(* Logix 5000 AddOnInstructionDefinition export MAG_Yaskawa; software revision 17.00 *)

TYPE Yaskawa_EIP_Servo :   // Yaskawa SigmaLogic Axis Structure v2.4.0
STRUCT
   O : Yaskawa_OUT_to_Servo;
   I : Yaskawa_IN_from_Servo;
   AOI_SB : Yaskawa_AOI_Status_Bits;
END_STRUCT
END_TYPE

TYPE Yaskawa_OUT_to_Servo :   // Structure of data sent out to the Yaskawa SigmaLogic controller v2.4.0
STRUCT
   b00_ServoOn : BOOL;   // Servo On
   b01_Stop : BOOL;   // Stops All Current Motion in Progress
   b02_Home : BOOL;   // Start Homing Process
   b03_MoveStart1 : BOOL;   // Start Current Motion
   b06_SuperImpose : BOOL;
   b07_ServoAlarmReset : BOOL;   // Servo Alarm Reset
   b08_ControllerAlarmReset : BOOL;   // SigmaLogic Alarm Reset
   b09_MoveStart2 : BOOL;   // Start Second Motion (Blended Move)
   b10_MoveAbort : BOOL;   // Abort Current Move
   b11_MovePause : BOOL;   // Pause Current Move
   b12_SeqPause : BOOL;   // Indexing Sequence Pause
   b13_SeqResume : BOOL;   // Indexing Sequence Resume
   b14_SeqCancel : BOOL;   // Indexing Sequence Cancel
   b15_AbsEncoderReset : BOOL;   // Absolute Encoder Reset
   b16_SeqStart : BOOL;   // Start Indexing Sequence
   b17_SeqEditSpeed : BOOL;   // Enter Edit Speed
   b18_SeqEditDistance : BOOL;   // Enter Distance Edit
   b19_PLSEnable : BOOL;   // Enable PLS execution
   b20_PLSActivateOutput1 : BOOL;   // Activate PLS output1 switch logic
   b21_PLSActivateOutput2 : BOOL;   // Activate PLS output2 switch logic
   b22_PLSActivateOutput3 : BOOL;   // Activate PLS output3 switch logic
   b23_PLSActivateOutput4 : BOOL;   // Activate PLS output4 switch logic
   b24_SetClock : BOOL;   // Set the remote controller clock with data provided by the PLC
   RebootController : BOOL;
   UseExternalEncoder : BOOL;   // Use External Encoder when executing MAHSP_Yaskawa
   b32_HeatbeatAnswer : BOOL;   // Heartbeat Answer
   BrakeBypassRequest : BOOL;
   SetFwdTorqueLimit : BOOL;
   SetRevTorqueLimit : BOOL;
   TorqueLimit : DINT;
   TorqueRamp : DINT;
   HomeMethod : INT;
   HomeSpeed : DINT;
   HomeAccDec : DINT;   // Home Move Acceleration/Deceleration Rate
   HomeBackOffDistance : DINT;
   HomeCreepSpeed : DINT;
   HomeCreepDistanceLimit : DINT;
   HomeCreepTimeLimit : DINT;
   HomeOffsetDistance : DINT;
   HomeOffsetSpeed : DINT;
   HomePostion : DINT;
   HomeTorque : DINT;
   HomeInputNo : DINT;
   HomeApproachTimeLimit : DINT;
   HomeApproachDistLimit : DINT;
   HomeDirection : INT;
   HomeSwitchMode : INT;
   MoveType : INT;
   MoveDirection : INT;
   MoveAccel1 : DINT;
   MoveAccel2 : DINT;
   MoveDecel1 : DINT;
   MoveDecel2 : DINT;
   MoveSpeed1 : DINT;
   MoveSpeed2 : DINT;
   MoveDistance1 : DINT;
   MoveDistance2 : DINT;
   MovePosition1 : DINT;
   MovePosition2 : DINT;
   RegistrationDistance : DINT;
   GearNumerator : DINT;
   GearDenominator : DINT;
   SuperImposeDistance : DINT;
   Resolution : INT;
   RegistrationDirection : INT;
   TuningLevel : INT;
   SequenceStep : INT;   // Staring Sequence Step Number
   SequenceEditStep : INT;   // Sequence Step Number to Edit
   FlagCommandBits1 : DINT;   // Flag Commands. 1..64 are General Flags, Bits 0..31 correspond to Flag 1..32
   FlagCommandBits2 : DINT;   // Flag Commands cont. 1..64 are General Flags, Bits 0..31 correspond to Flag 33..64
   DigitalOutCommandBits : DINT;   // Digital Output commands. Bits 0-7 correspond to CN13 Digital Outputs 0-7, used as Flag 73-80. Bits 8-10 correspond to CN1 Digital Outputs 0-2 used as Flag 88-90"
   SequenceEditSpeed : DINT;
   SequenceEditDistance : DINT;
   FeedRateOverride : INT;
   HSI_Enable : BOOL;
   HSI_MoveMode : BOOL;   // 0=Relative; 1=Moves per Cycle
   HSI_CalcMethod : BOOL;   // 0=Accel/Decel; 1=Time
   HSI_MoveDirection : BOOL;   // 0 = Negative; 1 = Positive
   HSI_TriggerFlag : INT;
   HSI_MovingFlag : INT;
   HSI_DwellingFlag : INT;
   HSI_DoneFlag : INT;
   HSI_MoveType : INT;   // 0=Single; 1=Repeat; 2=Repeat "x" times
   HSI_RepeatNumber : INT;
   HSI_Distance : DINT;
   HSI_Speed : DINT;
   HSI_Accel : DINT;
   HSI_MoveTime : DINT;
   HSI_DwellTime : DINT;
   PLS_OutputFlag1 : INT;
   PLS_OutputFlag2 : INT;
   PLS_OutputFlag3 : INT;
   PLS_OutputFlag4 : INT;
   PLS_OnPosition1 : DINT;
   PLS_OffPosition1 : DINT;
   PLS_OnPosition2 : DINT;
   PLS_OffPosition2 : DINT;
   PLS_OnPosition3 : DINT;
   PLS_OffPosition3 : DINT;
   PLS_OnPosition4 : DINT;
   PLS_OffPosition4 : DINT;
   PLS_OnCompensation1 : INT;
   PLS_OffCompensation1 : INT;
   PLS_OnCompensation2 : INT;
   PLS_OffCompensation2 : INT;
   PLS_OnCompensation3 : INT;
   PLS_OffCompensation3 : INT;
   PLS_OnCompensation4 : INT;
   PLS_OffCompensation4 : INT;
   RTC_Year : INT;
   RTC_Month : INT;
   RTC_Day : INT;
   RTC_Hour : INT;
   RTC_Min : INT;
   RTC_Sec : INT;
   StopDecel : DINT;
   AnalogOutput : INT;   // CN13, AO_01 [mV]
END_STRUCT
END_TYPE

TYPE Yaskawa_AOI_Status_Bits :   // Internal bits used to interlock Yaskawa AOI execution. v2.4.0
STRUCT
   MAM : BOOL;   // Move AOI Active
   MAJ : BOOL;   // Jog AOI Active
   MAB : BOOL;   // Blending AOI Active
   MAG : BOOL;   // Gearing AOI Active
   MAHSP : BOOL;   // Home SetPoint AOI Active
   MAH : BOOL;   // Homing AOI Active
   MSQE : BOOL;   // Sequence Edit AOI Active
   MSQR : BOOL;   // Sequence Run AOI Active
   MHSI : BOOL;   // High Speed Index AOI Active
   MSO : BOOL;   // Servo On
   MSF : BOOL;   // Servo Off
   MAFR : BOOL;   // Fault Reset
   MAS : BOOL;   // Servo Abort
   MTRQ : BOOL;   // Torque Mode Active
   MPLS : BOOL;   // PLS Active
   MCLK : BOOL;   // SetClock Active
   MSTL : BOOL;   // Set Torque Limit Active
   AOI_Permissive : BOOL;   // Permissive to Execute an AOI
END_STRUCT
END_TYPE

TYPE Yaskawa_IN_from_Servo :   // Structure of data coming from the Yaskawa SigmaLogic controller. v2.4.0
STRUCT
   AlarmText : STRING;   // ServoPack Alarm Code plus Text Description
   b00_Heartbeat : BOOL;
   b01_Alarm : BOOL;   // ServoPack Alarm
   b02_Warning : BOOL;   // ServoPack Warning
   b03_Ready : BOOL;   // ServoPack Ready
   b04_Enabled : BOOL;   // ServoPack Enabled ("Servo On")
   b05_StopComplete : BOOL;
   b06_HomeComplete : BOOL;
   b07_HomeBusy : BOOL;
   b08_HomeActive : BOOL;
   b09_HomeAborted : BOOL;
   b10_HomeError : BOOL;
   b11_MoveAbsComplete : BOOL;
   b12_MoveAbsBusy : BOOL;
   b13_MoveAbsActive : BOOL;
   b14_MoveAbsAborted : BOOL;
   b15_MoveAbsError : BOOL;
   b16_MoveRelComplete : BOOL;
   b17_MoveRelBusy : BOOL;
   b18_MoveRelActive : BOOL;
   b19_MoveRelAborted : BOOL;
   b20_MoveRelError : BOOL;
   b21_JogAtSpeed : BOOL;
   b22_JogBusy : BOOL;
   b23_JogActive : BOOL;
   b24_JogAborted : BOOL;
   b25_JogError : BOOL;
   b26_GearInSync : BOOL;
   b27_GearBusy : BOOL;
   b28_GearActive : BOOL;
   b29_GearAborted : BOOL;
   b30_GearError : BOOL;
   b32_MoveSuperComplete : BOOL;
   b33_MoveSuperBusy : BOOL;
   b34_MoveSuperActive : BOOL;
   b35_MoveSuperAborted : BOOL;
   b36_MoveSuperError : BOOL;
   b37_PowerCycleRequired : BOOL;
   b38_MoveBlend1Complete : BOOL;
   b39_MoveBlend1Busy : BOOL;
   b40_MoveBlend1Active : BOOL;
   b41_MoveBlend1Abort : BOOL;
   b42_MoveBlend1Error : BOOL;
   b43_MoveBlend2Complete : BOOL;
   b44_MoveBlend2Busy : BOOL;
   b45_MoveBlend2Active : BOOL;
   b46_MoveBlend2Abort : BOOL;
   b47_MoveBlend2Error : BOOL;
   b48_RegComplete : BOOL;
   b49_RegBusy : BOOL;
   b50_RegActive : BOOL;
   b51_RegAborted : BOOL;
   b52_RegError : BOOL;
   b53_ResetAbsEncoderActive : BOOL;
   b54_ResetAbsEncoderBusy : BOOL;
   b55_ResetAbsEncoderDone : BOOL;
   b56_ResetAbsEncoderError : BOOL;
   b57_SeqRunning : BOOL;
   b58_RegSensorNotReached : BOOL;
   b59_SeqEditError : BOOL;
   b60_SeqEditDone : BOOL;
   b61_TorqueAtTorque : BOOL;
   b62_TorqueBusy : BOOL;
   b63_TorqueActive : BOOL;
   b64_TorqueAborted : BOOL;
   b65_TorqueError : BOOL;
   b66_ControllerAlarm : BOOL;
   b67_ApplicationError : BOOL;
   b68_AxisAtStandStill : BOOL;
   b69_TestModeActive : BOOL;
   b70_ServoParamsOK : BOOL;
   b71_SetFwdTorqueLimitDone : BOOL;
   b72_SetRevTorqueLimitDone : BOOL;
   Position : DINT;
   Speed : DINT;
   Torque : DINT;
   HomeErrorID : INT;
   MoveAbsErrorID : INT;
   MoveRelErrorID : INT;
   JogErrorID : INT;
   GearErrorID : INT;
   MoveSuperErrorID : INT;
   ServoAlarmID : INT;
   ServoWarningID : INT;
   ControllerAlarmID : DINT;
   AxisGenAlarmID : DINT;
   MoveBlend1ErrorID : INT;
   MoveBlend2ErrorID : INT;
   ResetAbsEncoderErrorID : INT;
   FunctionBlockErrorID : INT;
   TorqueErrorID : INT;
   RegErrorID : INT;
   SeqCurrentStep : INT;
   FlagStatusBit1 : DINT;   // Flag Status. 1..64 are General Flags, Bits 0..31 correspond to Flag 1..32
   FlagStatusBit2 : DINT;   // Flag Status cont. 1..64 are General Flags, Bits 0..31 correspond to Flag 33..64
   IOStatusBits : DINT;   // Digital IO Status. Bits 0-7, CN13 Inputs 0-7, Used as Flag 65-72. Bits 8-15, CN13 Outputs 0-7, Used as Flag 73-80. Bits 16-22, CN1 Inputs 0-6, Used as Flag 81-87. Bits 23-25, CN1 Outputs 0-4, Used as Flag 88-92.
   HSI_Moving : BOOL;
   HSI_Dwelling : BOOL;
   HSI_Done : BOOL;
   HSI_Busy : BOOL;
   HSI_Error : BOOL;
   HSI_ErrorCode : INT;
   PLS_Running : BOOL;
   PLS_SwitchStatus1 : BOOL;
   PLS_SwitchStatus2 : BOOL;
   PLS_SwitchStatus3 : BOOL;
   PLS_SwitchStatus4 : BOOL;
   PLS_Busy : BOOL;
   PLS_Error : BOOL;
   PLS_ErrorCode : INT;
   SetClock_Done : BOOL;
   SetClock_Busy : BOOL;
   SetClock_Error : BOOL;
   SetClock_ErrorID : INT;
   SoftwareVersion : DINT;
   FirmwareVersion : DINT;
   CommandedPos : DINT;
   CommandedPosNonCyc : DINT;
   CommandedSpeed : DINT;
   Clock_Year : INT;
   Clock_Month : INT;
   Clock_Day : INT;
   Clock_Hour : INT;
   Clock_Minute : INT;
   Clock_Second : INT;
   AnalogInput : REAL;   // CN13, AI_01 [v]
   BrakeBypassActive : BOOL;
   ForwardTorqueLimit : DINT;
   ReverseTorqueLimit : DINT;
END_STRUCT
END_TYPE

ADD_ON_INSTRUCTION MAG_Yaskawa   (* revision 2.4 0, vendor Yaskawa America, Inc., ExecuteEnableInFalse *)
// Motion Axis Gear
// Revision note:
// 2.4.0: No functional change
// 2.3.1: No functional change
// 2.3.0: Fixed bug with exiting MAG properly. Needed to clear MoveType as part of the stopping process not after it was done.
// 2.0.0: Improved output operation and error code reporting. Improved interlocking with embedded code.
// 1.2.0: No functional change.
// Initial Release 9/10/2014
// Help:
// This AOI moves a servo axis in direct proportion to the external encoder at a specified gear ratio. If desired, Superimposed moves may be enabled and executed on top of the gearing motion to adjust the servo position with respect to the external encoder. Acceleration and deceleration is performed at a fixed rate and not over any particular external encoder travel distance. The distance traveled during acceleration will depend on the rate/ratio specified and the current speed of the external encoder. Gear ratio is specified as Slave_Counts/Master_Counts where the values are both DINTs.
VAR_IN_OUT
   Axis : Yaskawa_EIP_Servo; {required}
END_VAR
VAR_INPUT
   Direction : INT; {required}   // 0 = slave axis moves in the same direction as the master axis 1 = slave axis moves in the opposite direction of the master axis. 2 = slave axis reverses from its current or previous direction 3 = slave axis continues in its current or previous direction
   Slave_Counts : DINT; {required}   // Gear Ratio Numerator
   Master_Counts : DINT; {required}   // Gear Ratio Denominator
   Accel_Rate : REAL; {required}   // Acceleration for the Gearing IN [unit/s/s]
   Decel_Rate : REAL; {required}   // Deceleration for the Gearing OUT [unit/s/s]
   SuperUse : INT; {required}   // 0 = Do Not Use Superimpose on Gear 1 = Use SuperImpose on Gear .
   SuperStart : BOOL; {required}   // Signal (pulse) that Starts the SuperImposed Move
   SuperSpeed : REAL; {required}   // Commanded Speed for the SuperImposed Move [unit/s]
   SuperAccel : REAL; {required}   // Acceleration for the SuperImposed Move [unit/s/s]
   SuperDecel : REAL; {required}   // Deceleration for the SuperImposed Move [unit/s/s]
   SuperDistance : REAL; {required}   // Distance (Relative) for the SuperImposed Move [unit/s/s]
END_VAR
VAR_OUTPUT
   EN : BOOL; {visible}   // The AOI is Active
   DN : BOOL; {visible}   // Servo and External Gearing in Sync.
   IP : BOOL; {visible}   // Gearing is In Process
   ER : BOOL; {visible}   // Gearing Motion Error
   SDN : BOOL; {visible}   // SuperImposed Move is Finished
   SIP : BOOL; {visible}   // SuperImposed Move is In Process
   SER : BOOL; {visible}   // SuperImposed Move Error
   FLT_RDY : BOOL; {visible}   // The Servo is Not Ready
   FLT_BSY : BOOL; {visible}   // There is another AOI Active for this Axis
   GearErrorCode : INT; {visible}   // Gearing Error Code
   SuperErrorCode : INT; {visible}   // Move Superimposed Error Code
END_VAR
VAR
   AOI_ON_LOCAL : BOOL;
   db90 : BOOL;   // Shot90
   ScaleFactor : DINT;
   Execute_OS : BOOL;
   Stopping : BOOL;
   Finished : BOOL;   // Function is finished
END_VAR

ROUTINE EnableInFalse   (* ladder *)
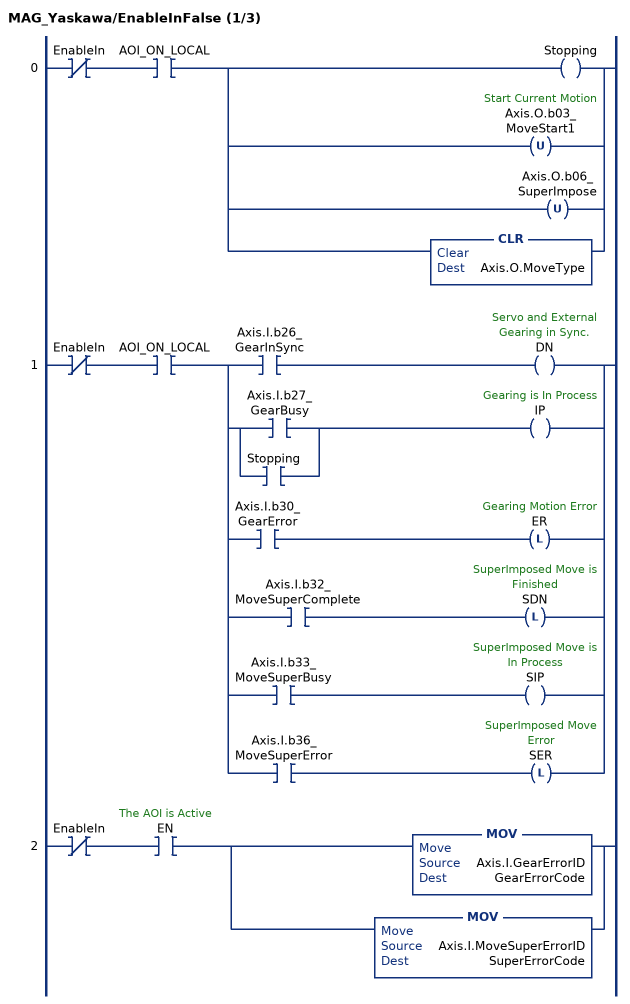
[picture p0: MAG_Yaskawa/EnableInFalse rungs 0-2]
   0: XIO(EnableIn)XIC(AOI_ON_LOCAL)[OTE(Stopping) ,OTU(Axis.O.b03_MoveStart1) ,OTU(Axis.O.b06_SuperImpose) ,CLR(Axis.O.MoveType) ];
   1: XIO(EnableIn)XIC(AOI_ON_LOCAL)[XIC(Axis.I.b26_GearInSync) OTE(DN) ,[XIC(Axis.I.b27_GearBusy) ,XIC(Stopping) ] OTE(IP) ,XIC(Axis.I.b30_GearError) OTL(ER) ,XIC(Axis.I.b32_MoveSuperComplete) OTL(SDN) ,XIC(Axis.I.b33_MoveSuperBusy) OTE(SIP) ,XIC(Axis.I.b36_MoveSuperError) OTL(SER) ];
   2: XIO(EnableIn)XIC(EN)[MOV(Axis.I.GearErrorID,GearErrorCode) ,MOV(Axis.I.MoveSuperErrorID,SuperErrorCode) ];
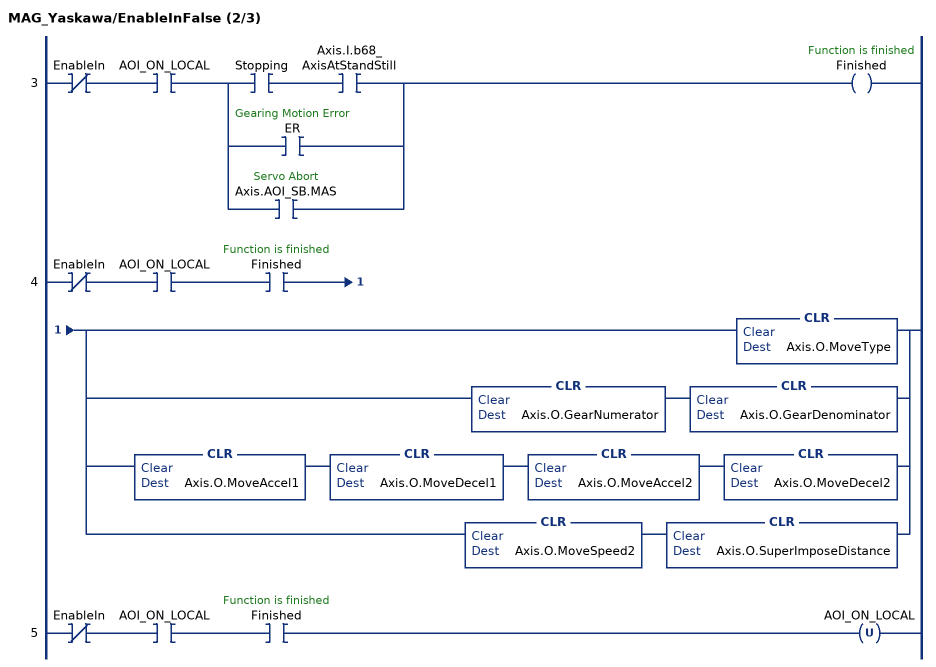
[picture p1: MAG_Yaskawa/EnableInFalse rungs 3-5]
   3: XIO(EnableIn)XIC(AOI_ON_LOCAL)[XIC(Stopping) XIC(Axis.I.b68_AxisAtStandStill) ,XIC(ER) ,XIC(Axis.AOI_SB.MAS) ]OTE(Finished);
   4: XIO(EnableIn)XIC(AOI_ON_LOCAL)XIC(Finished)[CLR(Axis.O.MoveType) ,CLR(Axis.O.GearNumerator) CLR(Axis.O.GearDenominator) ,CLR(Axis.O.MoveAccel1) CLR(Axis.O.MoveDecel1) CLR(Axis.O.MoveAccel2) CLR(Axis.O.MoveDecel2) ,CLR(Axis.O.MoveSpeed2) CLR(Axis.O.SuperImposeDistance) ];
   5: XIO(EnableIn)XIC(AOI_ON_LOCAL)XIC(Finished)OTU(AOI_ON_LOCAL);
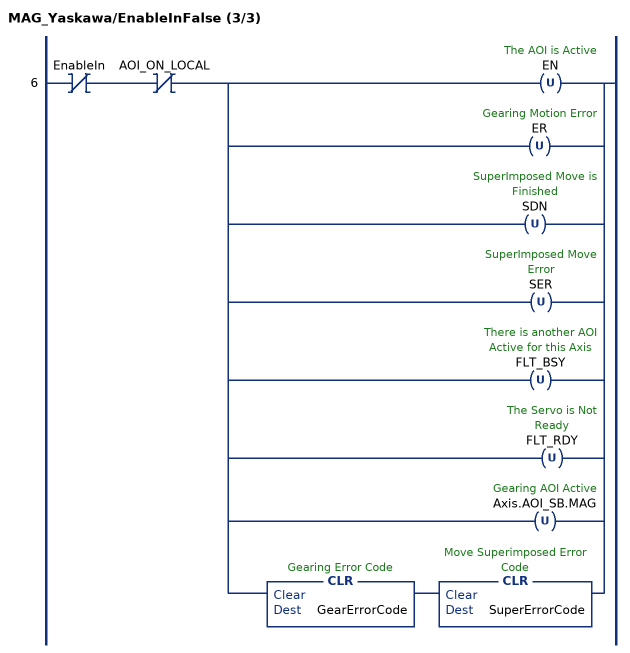
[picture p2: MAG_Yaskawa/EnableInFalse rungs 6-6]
   6: XIO(EnableIn)XIO(AOI_ON_LOCAL)[OTU(EN) ,OTU(ER) ,OTU(SDN) ,OTU(SER) ,OTU(FLT_BSY) ,OTU(FLT_RDY) ,OTU(Axis.AOI_SB.MAG) ,CLR(GearErrorCode) CLR(SuperErrorCode) ];
END_ROUTINE

ROUTINE Logic   (* ladder *)
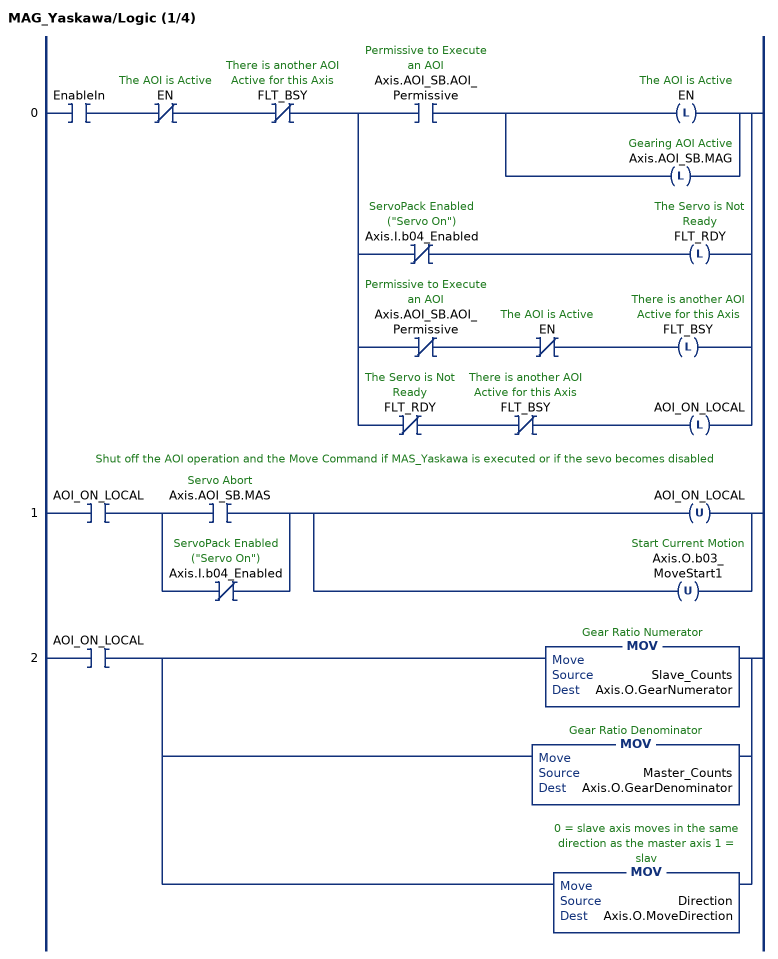
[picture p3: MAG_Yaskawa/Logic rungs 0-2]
   0: XIC(EnableIn)XIO(EN)XIO(FLT_BSY)[XIC(Axis.AOI_SB.AOI_Permissive) [OTL(EN) ,OTL(Axis.AOI_SB.MAG) ] ,XIO(Axis.I.b04_Enabled) OTL(FLT_RDY) ,XIO(Axis.AOI_SB.AOI_Permissive) XIO(EN) OTL(FLT_BSY) ,XIO(FLT_RDY) XIO(FLT_BSY) OTL(AOI_ON_LOCAL) ];
   // Shut off the AOI operation and the Move Command if MAS_Yaskawa is executed or if the sevo becomes disabled
   1: XIC(AOI_ON_LOCAL)[XIC(Axis.AOI_SB.MAS) ,XIO(Axis.I.b04_Enabled) ][OTU(AOI_ON_LOCAL) ,OTU(Axis.O.b03_MoveStart1) ];
   2: XIC(AOI_ON_LOCAL)[MOV(Slave_Counts,Axis.O.GearNumerator) ,MOV(Master_Counts,Axis.O.GearDenominator) ,MOV(Direction,Axis.O.MoveDirection) ];
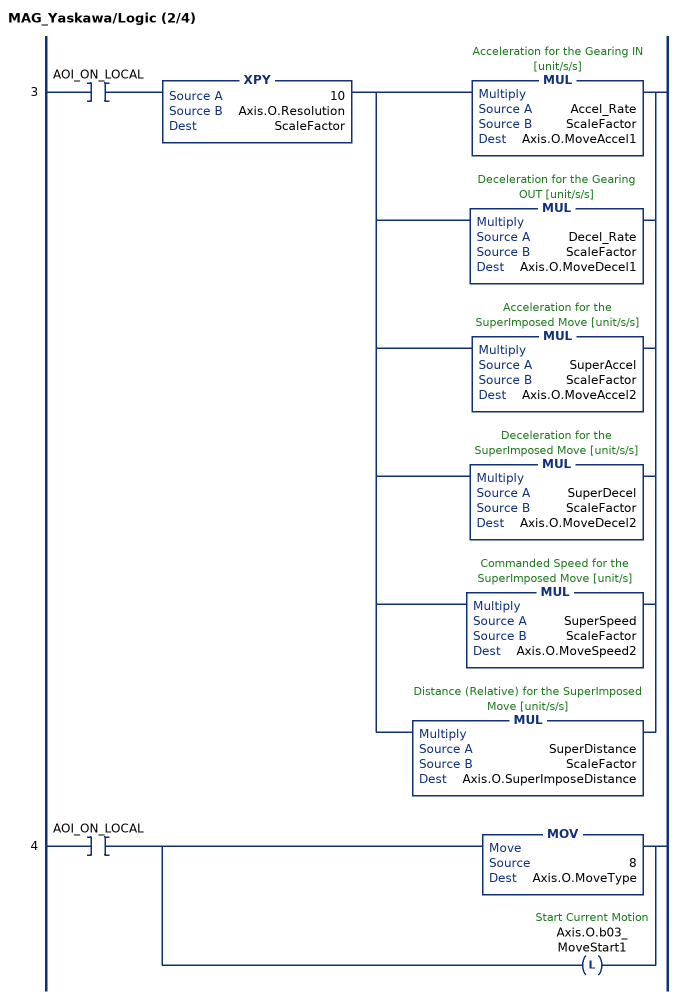
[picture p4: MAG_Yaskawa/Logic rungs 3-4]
   3: XIC(AOI_ON_LOCAL)XPY(10,Axis.O.Resolution,ScaleFactor)[MUL(Accel_Rate,ScaleFactor,Axis.O.MoveAccel1) ,MUL(Decel_Rate,ScaleFactor,Axis.O.MoveDecel1) ,MUL(SuperAccel,ScaleFactor,Axis.O.MoveAccel2) ,MUL(SuperDecel,ScaleFactor,Axis.O.MoveDecel2) ,MUL(SuperSpeed,ScaleFactor,Axis.O.MoveSpeed2) ,MUL(SuperDistance,ScaleFactor,Axis.O.SuperImposeDistance) ];
   4: XIC(AOI_ON_LOCAL)[MOV(8,Axis.O.MoveType) ,OTL(Axis.O.b03_MoveStart1) ];
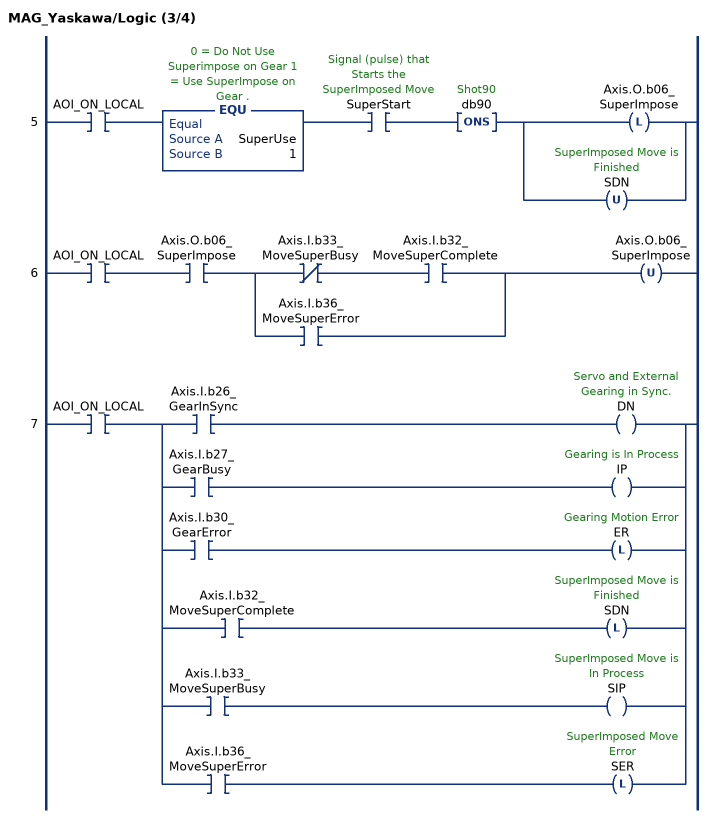
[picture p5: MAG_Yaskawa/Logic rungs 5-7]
   5: XIC(AOI_ON_LOCAL)EQU(SuperUse,1)XIC(SuperStart)ONS(db90)[OTL(Axis.O.b06_SuperImpose) ,OTU(SDN) ];
   6: XIC(AOI_ON_LOCAL)XIC(Axis.O.b06_SuperImpose)[XIO(Axis.I.b33_MoveSuperBusy) XIC(Axis.I.b32_MoveSuperComplete) ,XIC(Axis.I.b36_MoveSuperError) ]OTU(Axis.O.b06_SuperImpose);
   7: XIC(AOI_ON_LOCAL)[XIC(Axis.I.b26_GearInSync) OTE(DN) ,XIC(Axis.I.b27_GearBusy) OTE(IP) ,XIC(Axis.I.b30_GearError) OTL(ER) ,XIC(Axis.I.b32_MoveSuperComplete) OTL(SDN) ,XIC(Axis.I.b33_MoveSuperBusy) OTE(SIP) ,XIC(Axis.I.b36_MoveSuperError) OTL(SER) ];
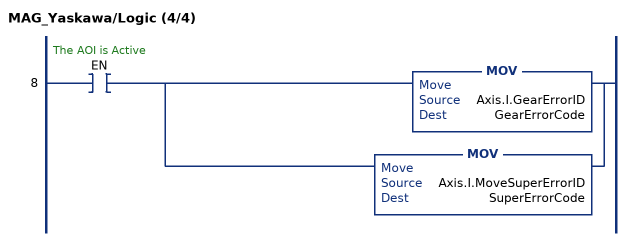
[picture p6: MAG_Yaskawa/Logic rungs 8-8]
   8: XIC(EN)[MOV(Axis.I.GearErrorID,GearErrorCode) ,MOV(Axis.I.MoveSuperErrorID,SuperErrorCode) ];
END_ROUTINE
END_ADD_ON_INSTRUCTION
